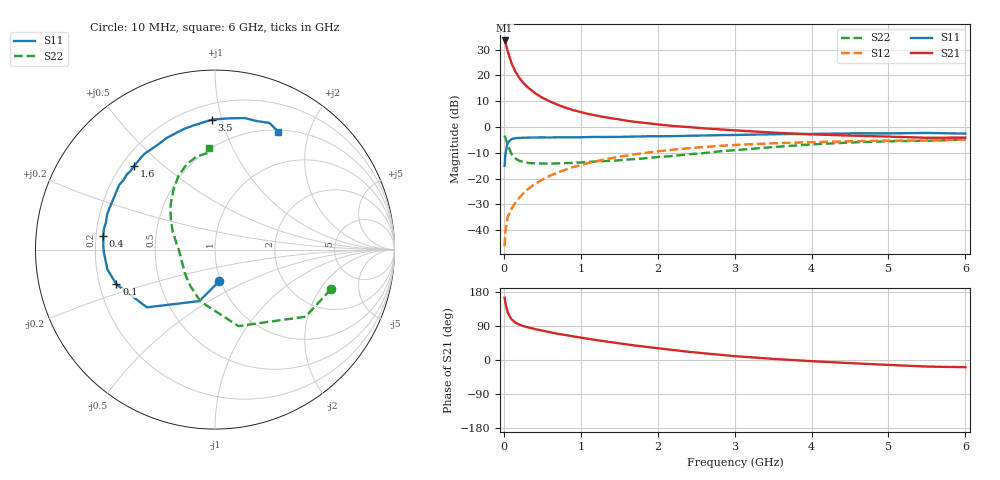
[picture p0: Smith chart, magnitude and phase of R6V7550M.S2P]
! SIEMENS Small Signal Semiconductors
! BFR193
! Si NPN RF Bipolar Junction Transistor in SOT23
! VCE = 0.75 V  IC = 50 mA
! Common Emitter S-Parameters:  May  1996
# GHz  S  MA  R  50
!  f  S11  S21  S12  S22
! GHz  MAG  ANG  MAG  ANG  MAG  ANG  MAG  ANG
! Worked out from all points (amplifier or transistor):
!   36 points, 10 MHz to 6 GHz, reference 50 ohm
!   highest |S21| = 33.6 dB at 10 MHz (marker M1)
!   |S21| within 3 dB of that: start of sweep to 39.54 MHz
!   unconditionally stable (mu >= 1): start of sweep to 11.79 MHz; 187.9 MHz to end of sweep
!   at 250 MHz: K = 1.05, MAG = 20.2 dB, |S12| = -25.8 dB
!   at 1.4 GHz: K = 1.07, MAG = 6.1 dB, |S12| = -12.1 dB
!   at 6 GHz: K = 1.02, MAG = -0.5 dB, |S12| = -4.8 dB
!   S11 on the Smith chart (normalised r, x): 10 MHz: 0.98, -0.36; 100 MHz: 0.27, -0.16; 400 MHz: 0.23, +0.06; 1.6 GHz: 0.25, +0.40; 3.5 GHz: 0.31, +0.93; 6 GHz: 0.52, +1.55
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0.01  0.1773 -82.4  47.66 164.4  0.0049 72.4  0.6824 -18.9
0.02  0.2993 -106.7  43.44 150.9  0.0094 65.7  0.6281 -36.5
0.05  0.4974 -139.7  29.47 125.1  0.0179 59.7  0.4457 -73.0
0.1  0.5822 -160.6  17.15 107.2  0.0262 61.9  0.2998 -105.6
0.15  0.6099 -169.6  11.88 98.7  0.0342 64.7  0.2464 -123.4
0.2  0.6132 -174.6  9.02 93.4  0.0425 68.0  0.2221 -135.5
0.25  0.6195 -178.7  7.24 89.6  0.0514 69.2  0.2109 -144.4
0.3  0.6224 178.5  6.087 86.8  0.0604 70.4  0.2024 -149.8
0.4  0.6275 172.9  4.601 81.8  0.0779 70.8  0.1969 -158.9
0.5  0.6295 169.4  3.698 77.6  0.0956 70.6  0.1961 -165.8
0.6  0.6263 165.6  3.119 73.3  0.1136 69.7  0.1957 -170.0
0.7  0.6321 162.0  2.703 69.2  0.1312 68.8  0.197 -173.3
0.9  0.6319 155.3  2.132 62.4  0.1665 65.8  0.2022 179.7
1.1  0.6389 148.8  1.791 55.8  0.2005 62.5  0.2109 175.1
1.3  0.6397 142.9  1.565 49.6  0.2337 58.9  0.2183 170.1
1.6  0.649 134.0  1.322 41.2  0.2799 53.6  0.2338 163.9
2.2  0.6655 118.6  1.049 26.4  0.3635 42.7  0.275 151.1
3  0.7015 100.1  0.862 10.2  0.4483 28.2  0.3548 133.9
3.5  0.7244 91.3  0.78 3.0  0.4831 20.0  0.4091 124.3
4.5  0.7513 77.2  0.682 -8.2  0.5301 6.2  0.5007 108.3
5.5  0.7682 66.7  0.618 -17.3  0.5464 -6.2  0.5427 92.8
6  0.7453 61.7  0.624 -19.0  0.5743 -10.0  0.5691 93.5
